(* Logix 5000 Rung export; software revision 33.00 *)

TYPE Banner_IOL_Device :
STRUCT
   Initial_Global_Read : BOOL;
   Command : SINT;
   Data : Banner_IOL_Device_Index;
   Reset : BOOL;
END_STRUCT
END_TYPE

TYPE Banner_IOL_Device_Index :
STRUCT
   Index : Banner_IOL_Device_SubIndex[39];
END_STRUCT
END_TYPE

TYPE Banner_IOL_Device_SubIndex :
STRUCT
   Sub : DINT[34];
END_STRUCT
END_TYPE

TYPE Banner_IOL_Rules :
STRUCT
   Byte_Pos : SINT;   // Byte Position to read from or write data to.
   Multi : SINT;   // Determines if a multiple byte length index is being accessed. Use 2 for 2 bytes length, 3 for 3 byte length, etc..
   BitControl : BOOL;   // 0=Standard byte contorl, 1=Bitwise packaging
   BitPos : SINT;   // Bit start position for operation
   BitValue : SINT;
   Sub_Index : SINT;
   Signed : SINT;   // 0=Unsigned, 1=Signed
END_STRUCT
END_TYPE

TYPE Banner_IOL_Rules_Array :
STRUCT
   Length : DINT;
   Settings : Banner_IOL_Rules_SettingsArray[39];
END_STRUCT
END_TYPE

TYPE Banner_IOL_Rules_SettingsArray :
STRUCT
   Index : DINT;
   Sub_Index : DINT;
   Num_Op : INT;   // Number of Operations to read/write Index.
   Total_Bytes : INT;
   RW : SINT;   // 0 = Read Only, 1 = Write Only, 2 = Read or Write
   Rules : Banner_IOL_Rules[34];   // Sub Index Position in IODD.
END_STRUCT
END_TYPE

VAR_GLOBAL   (* controller tags *)
   S4B_IOLM1_01 : Banner_IOL_Device;
        .DATA.INDEX[2]   // Direct Parameters 1 (ro)
        .DATA.INDEX[2].SUB[1]   // Reserved
        .DATA.INDEX[2].SUB[2]   // Master Cycle Time
        .DATA.INDEX[2].SUB[3]   // Min Cycle Time
        .DATA.INDEX[2].SUB[4]   // M Sequence Capability
        .DATA.INDEX[2].SUB[5]   // IO-Link Version ID
        .DATA.INDEX[2].SUB[6]   // Process Data Input Length
        .DATA.INDEX[2].SUB[7]   // Process Data Output Length
        .DATA.INDEX[2].SUB[8]   // Vendor ID
        .DATA.INDEX[2].SUB[9]   // Device ID
        .DATA.INDEX[3]   // Standard Command (wo)
        .DATA.INDEX[3].SUB[1]   // Standard Command: 126=Locator Start, 127=Locator Stop, 129=Application Reset, 164=Reset All Metrics
        .DATA.INDEX[4]   // Serial Number (ro)
        .DATA.INDEX[4].SUB[1]   // SN1
        .DATA.INDEX[4].SUB[2]   // SN2
        .DATA.INDEX[4].SUB[3]   // SN3
        .DATA.INDEX[4].SUB[4]   // SN4
        .DATA.INDEX[4].SUB[5]   // SN5
        .DATA.INDEX[4].SUB[6]   // SN6
        .DATA.INDEX[4].SUB[7]   // SN7
        .DATA.INDEX[4].SUB[8]   // SN8
        .DATA.INDEX[4].SUB[9]   // SN9
        .DATA.INDEX[4].SUB[10]   // SN10
        .DATA.INDEX[4].SUB[11]   // SN11
        .DATA.INDEX[4].SUB[12]   // SN12
        .DATA.INDEX[4].SUB[13]   // SN13
        .DATA.INDEX[4].SUB[14]   // SN14
        .DATA.INDEX[4].SUB[15]   // SN15
        .DATA.INDEX[4].SUB[16]   // SN16
        .DATA.INDEX[5]   // Configurable IO Pin Settings
        .DATA.INDEX[5].SUB[1]   // Pin Control: 0=Weak Beam, 1=Auxiliary Output, 2=Indicatoer Override Input, 3=Unused
        .DATA.INDEX[5].SUB[2]   // Control Type: 0=PNP, 1=NPN
        .DATA.INDEX[5].SUB[3]   // Indicator Override Host: 0=Enabled, 1=Disabled
        .DATA.INDEX[5].SUB[4]   // Indicator Override Guest 1: 0=Enabled, 1=Disabled
        .DATA.INDEX[5].SUB[5]   // Indicator Override Guest 2: 0=Enabled, 1=Disabled
        .DATA.INDEX[5].SUB[6]   // Indicator Override Guest 3: 0=Enabled, 1=Disabled
        .DATA.INDEX[6]   // All Curtains Clear Settings
        .DATA.INDEX[6].SUB[1]   // Endcap Color 1: 0=Green, 1=Red, 2=Yellow, 3=White, 4=Blue, 5=Magenta, 6=Cyan
        .DATA.INDEX[6].SUB[2]   // Endcap Intensity 1: 0=High, 1=Medium, 2=Low, 3=Off
        .DATA.INDEX[6].SUB[3]   // Endcap Animation Style: 0=Steady, 1=Flash, 2=Alternate
        .DATA.INDEX[6].SUB[4]   // Endcap Color 2: 0=Green, 1=Red, 2=Yellow, 3=White, 4=Blue, 5=Magenta, 6=Cyan
        .DATA.INDEX[6].SUB[5]   // Endcap Intensity 2: 0=High, 1=Medium, 2=Low, 3=Off
        .DATA.INDEX[6].SUB[6]   // Endcap Animation Speed: 0=Fast, 1=Medium, 2=Slow
        .DATA.INDEX[7]   // Any Curtain Weak Beam Settings
        .DATA.INDEX[7].SUB[1]   // Endcap Color 1: 0=Green, 1=Red, 2=Yellow, 3=White, 4=Blue, 5=Magenta, 6=Cyan
        .DATA.INDEX[7].SUB[2]   // Endcap Intensity 1: 0=High, 1=Medium, 2=Low, 3=Off
        .DATA.INDEX[7].SUB[3]   // Endcap Animation Style: 0=Steady, 1=Flash, 2=Alternate
        .DATA.INDEX[7].SUB[4]   // Endcap Color 2: 0=Green, 1=Red, 2=Yellow, 3=White, 4=Blue, 5=Magenta, 6=Cyan
        .DATA.INDEX[7].SUB[5]   // Endcap Intensity 2: 0=High, 1=Medium, 2=Low, 3=Off
        .DATA.INDEX[7].SUB[6]   // Endcap Animation Speed: 0=Fast, 1=Medium, 2=Slow
        .DATA.INDEX[8]   // This Curtain Weak Beam Settings
        .DATA.INDEX[8].SUB[1]   // Endcap Color 1: 0=Green, 1=Red, 2=Yellow, 3=White, 4=Blue, 5=Magenta, 6=Cyan
        .DATA.INDEX[8].SUB[2]   // Endcap Intensity 1: 0=High, 1=Medium, 2=Low, 3=Off
        .DATA.INDEX[8].SUB[3]   // Endcap Animation Style: 0=Steady, 1=Flash, 2=Alternate
        .DATA.INDEX[8].SUB[4]   // Endcap Color 2: 0=Green, 1=Red, 2=Yellow, 3=White, 4=Blue, 5=Magenta, 6=Cyan
        .DATA.INDEX[8].SUB[5]   // Endcap Intensity 2: 0=High, 1=Medium, 2=Low, 3=Off
        .DATA.INDEX[8].SUB[6]   // Endcap Animation Speed: 0=Fast, 1=Medium, 2=Slow
        .DATA.INDEX[9]   // Any Curtain Blocked Settings
        .DATA.INDEX[9].SUB[1]   // Endcap Color 1: 0=Green, 1=Red, 2=Yellow, 3=White, 4=Blue, 5=Magenta, 6=Cyan
        .DATA.INDEX[9].SUB[2]   // Endcap Intensity 1: 0=High, 1=Medium, 2=Low, 3=Off
        .DATA.INDEX[9].SUB[3]   // Endcap Animation Style: 0=Steady, 1=Flash, 2=Alternate
        .DATA.INDEX[9].SUB[4]   // Endcap Color 2: 0=Green, 1=Red, 2=Yellow, 3=White, 4=Blue, 5=Magenta, 6=Cyan
        .DATA.INDEX[9].SUB[5]   // Endcap Intensity 2: 0=High, 1=Medium, 2=Low, 3=Off
        .DATA.INDEX[9].SUB[6]   // Endcap Animation Speed: 0=Fast, 1=Medium, 2=Slow
        .DATA.INDEX[10]   // This Curtain Blocked Settings
        .DATA.INDEX[10].SUB[1]   // Endcap Color 1: 0=Green, 1=Red, 2=Yellow, 3=White, 4=Blue, 5=Magenta, 6=Cyan
        .DATA.INDEX[10].SUB[2]   // Endcap Intensity 1: 0=High, 1=Medium, 2=Low, 3=Off
        .DATA.INDEX[10].SUB[3]   // Endcap Animation Style: 0=Steady, 1=Flash, 2=Alternate
        .DATA.INDEX[10].SUB[4]   // Endcap Color 2: 0=Green, 1=Red, 2=Yellow, 3=White, 4=Blue, 5=Magenta, 6=Cyan
        .DATA.INDEX[10].SUB[5]   // Endcap Intensity 2: 0=High, 1=Medium, 2=Low, 3=Off
        .DATA.INDEX[10].SUB[6]   // Endcap Animation Speed: 0=Fast, 1=Medium, 2=Slow
        .DATA.INDEX[11]   // Indicator Override Input Settings
        .DATA.INDEX[11].SUB[1]   // Endcap Color 1: 0=Green, 1=Red, 2=Yellow, 3=White, 4=Blue, 5=Magenta, 6=Cyan
        .DATA.INDEX[11].SUB[2]   // Endcap Intensity 1: 0=High, 1=Medium, 2=Low, 3=Off
        .DATA.INDEX[11].SUB[3]   // Endcap Animation Style: 0=Steady, 1=Flash, 2=Alternate
        .DATA.INDEX[11].SUB[4]   // Endcap Color 2: 0=Green, 1=Red, 2=Yellow, 3=White, 4=Blue, 5=Magenta, 6=Cyan
        .DATA.INDEX[11].SUB[5]   // Endcap Intensity 2: 0=High, 1=Medium, 2=Low, 3=Off
        .DATA.INDEX[11].SUB[6]   // Endcap Animation Speed: 0=Fast, 1=Medium, 2=Slow
        .DATA.INDEX[12]   // Indicator Override IOL 1 Settings
        .DATA.INDEX[12].SUB[1]   // Endcap Color 1: 0=Green, 1=Red, 2=Yellow, 3=White, 4=Blue, 5=Magenta, 6=Cyan
        .DATA.INDEX[12].SUB[2]   // Endcap Intensity 1: 0=High, 1=Medium, 2=Low, 3=Off
        .DATA.INDEX[12].SUB[3]   // Endcap Animation Style: 0=Steady, 1=Flash, 2=Alternate
        .DATA.INDEX[12].SUB[4]   // Endcap Color 2: 0=Green, 1=Red, 2=Yellow, 3=White, 4=Blue, 5=Magenta, 6=Cyan
        .DATA.INDEX[12].SUB[5]   // Endcap Intensity 2: 0=High, 1=Medium, 2=Low, 3=Off
        .DATA.INDEX[12].SUB[6]   // Endcap Animation Speed: 0=Fast, 1=Medium, 2=Slow
        .DATA.INDEX[13]   // Indicator Override IOL 2 Settings
        .DATA.INDEX[13].SUB[1]   // Endcap Color 1: 0=Green, 1=Red, 2=Yellow, 3=White, 4=Blue, 5=Magenta, 6=Cyan
        .DATA.INDEX[13].SUB[2]   // Endcap Intensity 1: 0=High, 1=Medium, 2=Low, 3=Off
        .DATA.INDEX[13].SUB[3]   // Endcap Animation Style: 0=Steady, 1=Flash, 2=Alternate
        .DATA.INDEX[13].SUB[4]   // Endcap Color 2: 0=Green, 1=Red, 2=Yellow, 3=White, 4=Blue, 5=Magenta, 6=Cyan
        .DATA.INDEX[13].SUB[5]   // Endcap Intensity 2: 0=High, 1=Medium, 2=Low, 3=Off
        .DATA.INDEX[13].SUB[6]   // Endcap Animation Speed: 0=Fast, 1=Medium, 2=Slow
        .DATA.INDEX[14]   // Indicator Override IOL 3 Settings
        .DATA.INDEX[14].SUB[1]   // Endcap Color 1: 0=Green, 1=Red, 2=Yellow, 3=White, 4=Blue, 5=Magenta, 6=Cyan
        .DATA.INDEX[14].SUB[2]   // Endcap Intensity 1: 0=High, 1=Medium, 2=Low, 3=Off
        .DATA.INDEX[14].SUB[3]   // Endcap Animation Style: 0=Steady, 1=Flash, 2=Alternate
        .DATA.INDEX[14].SUB[4]   // Endcap Color 2: 0=Green, 1=Red, 2=Yellow, 3=White, 4=Blue, 5=Magenta, 6=Cyan
        .DATA.INDEX[14].SUB[5]   // Endcap Intensity 2: 0=High, 1=Medium, 2=Low, 3=Off
        .DATA.INDEX[14].SUB[6]   // Endcap Animation Speed: 0=Fast, 1=Medium, 2=Slow
        .DATA.INDEX[15]   // Indicator Override IOL 4 Settings
        .DATA.INDEX[15].SUB[1]   // Endcap Color 1: 0=Green, 1=Red, 2=Yellow, 3=White, 4=Blue, 5=Magenta, 6=Cyan
        .DATA.INDEX[15].SUB[2]   // Endcap Intensity 1: 0=High, 1=Medium, 2=Low, 3=Off
        .DATA.INDEX[15].SUB[3]   // Endcap Animation Style: 0=Steady, 1=Flash, 2=Alternate
        .DATA.INDEX[15].SUB[4]   // Endcap Color 2: 0=Green, 1=Red, 2=Yellow, 3=White, 4=Blue, 5=Magenta, 6=Cyan
        .DATA.INDEX[15].SUB[5]   // Endcap Intensity 2: 0=High, 1=Medium, 2=Low, 3=Off
        .DATA.INDEX[15].SUB[6]   // Endcap Animation Speed: 0=Fast, 1=Medium, 2=Slow
        .DATA.INDEX[16]   // Indicator Override IOL 5 Settings
        .DATA.INDEX[16].SUB[1]   // Endcap Color 1: 0=Green, 1=Red, 2=Yellow, 3=White, 4=Blue, 5=Magenta, 6=Cyan
        .DATA.INDEX[16].SUB[2]   // Endcap Intensity 1: 0=High, 1=Medium, 2=Low, 3=Off
        .DATA.INDEX[16].SUB[3]   // Endcap Animation Style: 0=Steady, 1=Flash, 2=Alternate
        .DATA.INDEX[16].SUB[4]   // Endcap Color 2: 0=Green, 1=Red, 2=Yellow, 3=White, 4=Blue, 5=Magenta, 6=Cyan
        .DATA.INDEX[16].SUB[5]   // Endcap Intensity 2: 0=High, 1=Medium, 2=Low, 3=Off
        .DATA.INDEX[16].SUB[6]   // Endcap Animation Speed: 0=Fast, 1=Medium, 2=Slow
        .DATA.INDEX[17]   // Indicator Override IOL 6 Settings
        .DATA.INDEX[17].SUB[1]   // Endcap Color 1: 0=Green, 1=Red, 2=Yellow, 3=White, 4=Blue, 5=Magenta, 6=Cyan
        .DATA.INDEX[17].SUB[2]   // Endcap Intensity 1: 0=High, 1=Medium, 2=Low, 3=Off
        .DATA.INDEX[17].SUB[3]   // Endcap Animation Style: 0=Steady, 1=Flash, 2=Alternate
        .DATA.INDEX[17].SUB[4]   // Endcap Color 2: 0=Green, 1=Red, 2=Yellow, 3=White, 4=Blue, 5=Magenta, 6=Cyan
        .DATA.INDEX[17].SUB[5]   // Endcap Intensity 2: 0=High, 1=Medium, 2=Low, 3=Off
        .DATA.INDEX[17].SUB[6]   // Endcap Animation Speed: 0=Fast, 1=Medium, 2=Slow
        .DATA.INDEX[18]   // Indicator Override IOL 7 Settings
        .DATA.INDEX[18].SUB[1]   // Endcap Color 1: 0=Green, 1=Red, 2=Yellow, 3=White, 4=Blue, 5=Magenta, 6=Cyan
        .DATA.INDEX[18].SUB[2]   // Endcap Intensity 1: 0=High, 1=Medium, 2=Low, 3=Off
        .DATA.INDEX[18].SUB[3]   // Endcap Animation Style: 0=Steady, 1=Flash, 2=Alternate
        .DATA.INDEX[18].SUB[4]   // Endcap Color 2: 0=Green, 1=Red, 2=Yellow, 3=White, 4=Blue, 5=Magenta, 6=Cyan
        .DATA.INDEX[18].SUB[5]   // Endcap Intensity 2: 0=High, 1=Medium, 2=Low, 3=Off
        .DATA.INDEX[18].SUB[6]   // Endcap Animation Speed: 0=Fast, 1=Medium, 2=Slow
        .DATA.INDEX[19]   // Indicator Override IOL 8 Settings
        .DATA.INDEX[19].SUB[1]   // Endcap Color 1: 0=Green, 1=Red, 2=Yellow, 3=White, 4=Blue, 5=Magenta, 6=Cyan
        .DATA.INDEX[19].SUB[2]   // Endcap Intensity 1: 0=High, 1=Medium, 2=Low, 3=Off
        .DATA.INDEX[19].SUB[3]   // Endcap Animation Style: 0=Steady, 1=Flash, 2=Alternate
        .DATA.INDEX[19].SUB[4]   // Endcap Color 2: 0=Green, 1=Red, 2=Yellow, 3=White, 4=Blue, 5=Magenta, 6=Cyan
        .DATA.INDEX[19].SUB[5]   // Endcap Intensity 2: 0=High, 1=Medium, 2=Low, 3=Off
        .DATA.INDEX[19].SUB[6]   // Endcap Animation Speed: 0=Fast, 1=Medium, 2=Slow
        .DATA.INDEX[20]   // Indicator Override IOL 9 Settings
        .DATA.INDEX[20].SUB[1]   // Endcap Color 1: 0=Green, 1=Red, 2=Yellow, 3=White, 4=Blue, 5=Magenta, 6=Cyan
        .DATA.INDEX[20].SUB[2]   // Endcap Intensity 1: 0=High, 1=Medium, 2=Low, 3=Off
        .DATA.INDEX[20].SUB[3]   // Endcap Animation Style: 0=Steady, 1=Flash, 2=Alternate
        .DATA.INDEX[20].SUB[4]   // Endcap Color 2: 0=Green, 1=Red, 2=Yellow, 3=White, 4=Blue, 5=Magenta, 6=Cyan
        .DATA.INDEX[20].SUB[5]   // Endcap Intensity 2: 0=High, 1=Medium, 2=Low, 3=Off
        .DATA.INDEX[20].SUB[6]   // Endcap Animation Speed: 0=Fast, 1=Medium, 2=Slow
        .DATA.INDEX[21]   // Fault Lockout Settings
        .DATA.INDEX[21].SUB[1]   // Endcap Color 1: 0=Green, 1=Red, 2=Yellow, 3=White, 4=Blue, 5=Magenta, 6=Cyan
        .DATA.INDEX[21].SUB[2]   // Endcap Intensity 1: 0=High, 1=Medium, 2=Low, 3=Off
        .DATA.INDEX[21].SUB[3]   // Endcap Animation Style: 0=Steady, 1=Flash, 2=Alternate
        .DATA.INDEX[21].SUB[4]   // Endcap Color 2: 0=Green, 1=Red, 2=Yellow, 3=White, 4=Blue, 5=Magenta, 6=Cyan
        .DATA.INDEX[21].SUB[5]   // Endcap Intensity 2: 0=High, 1=Medium, 2=Low, 3=Off
        .DATA.INDEX[21].SUB[6]   // Endcap Animation Speed: 0=Fast, 1=Medium, 2=Slow
        .DATA.INDEX[22]   // Lockout 1 (ro)
        .DATA.INDEX[22].SUB[1]   // Lockout Condition: 0 to 65535
        .DATA.INDEX[22].SUB[2]   // Sub Code: 0 to 65535
        .DATA.INDEX[22].SUB[3]   // Instance: 0 to 65535
        .DATA.INDEX[22].SUB[4]   // Source Module: 0=Host, 1=Guest 1, 2=Guest 2, 3=Guest 3
        .DATA.INDEX[22].SUB[5]   // Source Micro: 0=Micro A, 1=Micro B
        .DATA.INDEX[23]   // Lockout 2 (ro)
        .DATA.INDEX[23].SUB[1]   // Lockout Condition: 0 to 65535
        .DATA.INDEX[23].SUB[2]   // Sub Code: 0 to 65535
        .DATA.INDEX[23].SUB[3]   // Instance: 0 to 65535
        .DATA.INDEX[23].SUB[4]   // Source Module: 0=Host, 1=Guest 1, 2=Guest 2, 3=Guest 3
        .DATA.INDEX[23].SUB[5]   // Source Micro: 0=Micro A, 1=Micro B
        .DATA.INDEX[24]   // Lockout 3 (ro)
        .DATA.INDEX[24].SUB[1]   // Lockout Condition: 0 to 65535
        .DATA.INDEX[24].SUB[2]   // Sub Code: 0 to 65535
        .DATA.INDEX[24].SUB[3]   // Instance: 0 to 65535
        .DATA.INDEX[24].SUB[4]   // Source Module: 0=Host, 1=Guest 1, 2=Guest 2, 3=Guest 3
        .DATA.INDEX[24].SUB[5]   // Source Micro: 0=Micro A, 1=Micro B
        .DATA.INDEX[25]   // Lockout 4 (ro)
        .DATA.INDEX[25].SUB[1]   // Lockout Condition: 0 to 65535
        .DATA.INDEX[25].SUB[2]   // Sub Code: 0 to 65535
        .DATA.INDEX[25].SUB[3]   // Instance: 0 to 65535
        .DATA.INDEX[25].SUB[4]   // Source Module: 0=Host, 1=Guest 1, 2=Guest 2, 3=Guest 3
        .DATA.INDEX[25].SUB[5]   // Source Micro: 0=Micro A, 1=Micro B
        .DATA.INDEX[26]   // Lockout 5 (ro)
        .DATA.INDEX[26].SUB[1]   // Lockout Condition: 0 to 65535
        .DATA.INDEX[26].SUB[2]   // Sub Code: 0 to 65535
        .DATA.INDEX[26].SUB[3]   // Instance: 0 to 65535
        .DATA.INDEX[26].SUB[4]   // Source Module: 0=Host, 1=Guest 1, 2=Guest 2, 3=Guest 3
        .DATA.INDEX[26].SUB[5]   // Source Micro: 0=Micro A, 1=Micro B
        .DATA.INDEX[27]   // Lockout 6 (ro)
        .DATA.INDEX[27].SUB[1]   // Lockout Condition: 0 to 65535
        .DATA.INDEX[27].SUB[2]   // Sub Code: 0 to 65535
        .DATA.INDEX[27].SUB[3]   // Instance: 0 to 65535
        .DATA.INDEX[27].SUB[4]   // Source Module: 0=Host, 1=Guest 1, 2=Guest 2, 3=Guest 3
        .DATA.INDEX[27].SUB[5]   // Source Micro: 0=Micro A, 1=Micro B
        .DATA.INDEX[28]   // Lockout 7 (ro)
        .DATA.INDEX[28].SUB[1]   // Lockout Condition: 0 to 65535
        .DATA.INDEX[28].SUB[2]   // Sub Code: 0 to 65535
        .DATA.INDEX[28].SUB[3]   // Instance: 0 to 65535
        .DATA.INDEX[28].SUB[4]   // Source Module: 0=Host, 1=Guest 1, 2=Guest 2, 3=Guest 3
        .DATA.INDEX[28].SUB[5]   // Source Micro: 0=Micro A, 1=Micro B
        .DATA.INDEX[29]   // Lockout 8 (ro)
        .DATA.INDEX[29].SUB[1]   // Lockout Condition: 0 to 65535
        .DATA.INDEX[29].SUB[2]   // Sub Code: 0 to 65535
        .DATA.INDEX[29].SUB[3]   // Instance: 0 to 65535
        .DATA.INDEX[29].SUB[4]   // Source Module: 0=Host, 1=Guest 1, 2=Guest 2, 3=Guest 3
        .DATA.INDEX[29].SUB[5]   // Source Micro: 0=Micro A, 1=Micro B
        .DATA.INDEX[30]   // Lockout 9 (ro)
        .DATA.INDEX[30].SUB[1]   // Lockout Condition: 0 to 65535
        .DATA.INDEX[30].SUB[2]   // Sub Code: 0 to 65535
        .DATA.INDEX[30].SUB[3]   // Instance: 0 to 65535
        .DATA.INDEX[30].SUB[4]   // Source Module: 0=Host, 1=Guest 1, 2=Guest 2, 3=Guest 3
        .DATA.INDEX[30].SUB[5]   // Source Micro: 0=Micro A, 1=Micro B
        .DATA.INDEX[31]   // Lockout 10 (ro)
        .DATA.INDEX[31].SUB[1]   // Lockout Condition: 0 to 65535
        .DATA.INDEX[31].SUB[2]   // Sub Code: 0 to 65535
        .DATA.INDEX[31].SUB[3]   // Instance: 0 to 65535
        .DATA.INDEX[31].SUB[4]   // Source Module: 0=Host, 1=Guest 1, 2=Guest 2, 3=Guest 3
        .DATA.INDEX[31].SUB[5]   // Source Micro: 0=Micro A, 1=Micro B
        .DATA.INDEX[32]   // Host Safety Firmware Version (ro)
        .DATA.INDEX[32].SUB[1]   // Firmware 1
        .DATA.INDEX[32].SUB[2]   // Firmware 2
        .DATA.INDEX[32].SUB[3]   // Firmware 3
        .DATA.INDEX[32].SUB[4]   // Firmware 4
        .DATA.INDEX[32].SUB[5]   // Firmware 5
        .DATA.INDEX[32].SUB[6]   // Firmware 6
        .DATA.INDEX[32].SUB[7]   // Firmware 7
        .DATA.INDEX[32].SUB[8]   // Firmware 8
        .DATA.INDEX[33]   // Guest 1 Safety Firmware Version (ro)
        .DATA.INDEX[33].SUB[1]   // Firmware 1
        .DATA.INDEX[33].SUB[2]   // Firmware 2
        .DATA.INDEX[33].SUB[3]   // Firmware 3
        .DATA.INDEX[33].SUB[4]   // Firmware 4
        .DATA.INDEX[33].SUB[5]   // Firmware 5
        .DATA.INDEX[33].SUB[6]   // Firmware 6
        .DATA.INDEX[33].SUB[7]   // Firmware 7
        .DATA.INDEX[33].SUB[8]   // Firmware 8
        .DATA.INDEX[34]   // Guest 2 Safety Firmware Version (ro)
        .DATA.INDEX[34].SUB[1]   // Firmware 1
        .DATA.INDEX[34].SUB[2]   // Firmware 2
        .DATA.INDEX[34].SUB[3]   // Firmware 3
        .DATA.INDEX[34].SUB[4]   // Firmware 4
        .DATA.INDEX[34].SUB[5]   // Firmware 5
        .DATA.INDEX[34].SUB[6]   // Firmware 6
        .DATA.INDEX[34].SUB[7]   // Firmware 7
        .DATA.INDEX[34].SUB[8]   // Firmware 8
        .DATA.INDEX[35]   // Guest 3 Safety Firmware Version (ro)
        .DATA.INDEX[35].SUB[1]   // Firmware 1
        .DATA.INDEX[35].SUB[2]   // Firmware 2
        .DATA.INDEX[35].SUB[3]   // Firmware 3
        .DATA.INDEX[35].SUB[4]   // Firmware 4
        .DATA.INDEX[35].SUB[5]   // Firmware 5
        .DATA.INDEX[35].SUB[6]   // Firmware 6
        .DATA.INDEX[35].SUB[7]   // Firmware 7
        .DATA.INDEX[35].SUB[8]   // Firmware 8
        .DATA.INDEX[36]   // Number of Channels per Stick (ro)
        .DATA.INDEX[36].SUB[1]   // Number of Channels on Host
        .DATA.INDEX[36].SUB[2]   // Number of Channels on Guest 1
        .DATA.INDEX[36].SUB[3]   // Number of Channels on Guest 2
        .DATA.INDEX[36].SUB[4]   // Number of Channels on Guest 3
   S4B_Rules : Banner_IOL_Rules_Array;
        .SETTINGS[2]   // Direct Parameters 1
        .SETTINGS[2].RULES[0]   // Reserved
        .SETTINGS[2].RULES[1]   // Master Cycle Time
        .SETTINGS[2].RULES[2]   // Min Cycle Time
        .SETTINGS[2].RULES[3]   // M-Sequence Capability
        .SETTINGS[2].RULES[4]   // IO-Link ID
        .SETTINGS[2].RULES[5]   // Process Data Input Length
        .SETTINGS[2].RULES[6]   // Process Data Output Length
        .SETTINGS[2].RULES[7]   // Vendor ID
        .SETTINGS[2].RULES[8]   // Device ID
        .SETTINGS[3]   // Standard Command
        .SETTINGS[3].RULES[0]   // Standard Command
        .SETTINGS[4]   // Serial Number
        .SETTINGS[4].RULES[0]   // SN1
        .SETTINGS[4].RULES[1]   // SN2
        .SETTINGS[4].RULES[2]   // SN3
        .SETTINGS[4].RULES[3]   // SN4
        .SETTINGS[4].RULES[4]   // SN5
        .SETTINGS[4].RULES[5]   // SN6
        .SETTINGS[4].RULES[6]   // SN7
        .SETTINGS[4].RULES[7]   // SN8
        .SETTINGS[4].RULES[8]   // SN9
        .SETTINGS[4].RULES[9]   // SN10
        .SETTINGS[4].RULES[10]   // SN11
        .SETTINGS[4].RULES[11]   // SN12
        .SETTINGS[4].RULES[12]   // SN13
        .SETTINGS[4].RULES[13]   // SN14
        .SETTINGS[4].RULES[14]   // SN15
        .SETTINGS[4].RULES[15]   // SN16
        .SETTINGS[5]   // Configuration IO Pin Settings
        .SETTINGS[5].RULES[0]   // Pin Control
        .SETTINGS[5].RULES[1]   // Control Type
        .SETTINGS[5].RULES[2]   // Indicator Override Host
        .SETTINGS[5].RULES[3]   // Indicator Override Guest 1
        .SETTINGS[5].RULES[4]   // Indicator Override Guest 2
        .SETTINGS[5].RULES[5]   // Indicator Override Guest 3
        .SETTINGS[6]   // All Curtains Clear Settings
        .SETTINGS[6].RULES[0]   // Endcap Color 1
        .SETTINGS[6].RULES[1]   // Endcap Intensity 1
        .SETTINGS[6].RULES[2]   // Endcap Animation Style
        .SETTINGS[6].RULES[3]   // Endcap Color 2
        .SETTINGS[6].RULES[4]   // Endcap Intensity 2
        .SETTINGS[6].RULES[5]   // Endcap Animation Speed
        .SETTINGS[7]   // Any Curtain Weak Beam Settings
        .SETTINGS[7].RULES[0]   // Endcap Color 1
        .SETTINGS[7].RULES[1]   // Endcap Intensity 1
        .SETTINGS[7].RULES[2]   // Endcap Animation Style
        .SETTINGS[7].RULES[3]   // Endcap Color 2
        .SETTINGS[7].RULES[4]   // Endcap Intensity 2
        .SETTINGS[7].RULES[5]   // Endcap Animation Speed
        .SETTINGS[8]   // This Curtain Weak Beam Settings
        .SETTINGS[8].RULES[0]   // Endcap Color 1
        .SETTINGS[8].RULES[1]   // Endcap Intensity 1
        .SETTINGS[8].RULES[2]   // Endcap Animation Style
        .SETTINGS[8].RULES[3]   // Endcap Color 2
        .SETTINGS[8].RULES[4]   // Endcap Intensity 2
        .SETTINGS[8].RULES[5]   // Endcap Animation Speed
        .SETTINGS[9]   // Any Curtain Blocked Settings
        .SETTINGS[9].RULES[0]   // Endcap Color 1
        .SETTINGS[9].RULES[1]   // Endcap Intensity 1
        .SETTINGS[9].RULES[2]   // Endcap Animation Style
        .SETTINGS[9].RULES[3]   // Endcap Color 2
        .SETTINGS[9].RULES[4]   // Endcap Intensity 2
        .SETTINGS[9].RULES[5]   // Endcap Animation Speed
        .SETTINGS[10]   // This Curtain Blocked Settings
        .SETTINGS[10].RULES[0]   // Endcap Color 1
        .SETTINGS[10].RULES[1]   // Endcap Intensity 1
        .SETTINGS[10].RULES[2]   // Endcap Animation Style
        .SETTINGS[10].RULES[3]   // Endcap Color 2
        .SETTINGS[10].RULES[4]   // Endcap Intensity 2
        .SETTINGS[10].RULES[5]   // Endcap Animation Speed
        .SETTINGS[11]   // Indicator Override Input Settings
        .SETTINGS[11].RULES[0]   // Endcap Color 1
        .SETTINGS[11].RULES[1]   // Endcap Intensity 1
        .SETTINGS[11].RULES[2]   // Endcap Animation Style
        .SETTINGS[11].RULES[3]   // Endcap Color 2
        .SETTINGS[11].RULES[4]   // Endcap Intensity 2
        .SETTINGS[11].RULES[5]   // Endcap Animation Speed
        .SETTINGS[12]   // Indicator Override IOL 1 Settings
        .SETTINGS[12].RULES[0]   // Endcap Color 1
        .SETTINGS[12].RULES[1]   // Endcap Intensity 1
        .SETTINGS[12].RULES[2]   // Endcap Animation Style
        .SETTINGS[12].RULES[3]   // Endcap Color 2
        .SETTINGS[12].RULES[4]   // Endcap Intensity 2
        .SETTINGS[12].RULES[5]   // Endcap Animation Speed
        .SETTINGS[13]   // Indicator Override IOL 2 Settings
        .SETTINGS[13].RULES[0]   // Endcap Color 1
        .SETTINGS[13].RULES[1]   // Endcap Intensity 1
        .SETTINGS[13].RULES[2]   // Endcap Animation Style
        .SETTINGS[13].RULES[3]   // Endcap Color 2
        .SETTINGS[13].RULES[4]   // Encap Intensity 2
        .SETTINGS[13].RULES[5]   // Encap Animation Speed
        .SETTINGS[14]   // Indicator Override IOL 3 Settings
        .SETTINGS[14].RULES[0]   // Endcap Color 1
        .SETTINGS[14].RULES[1]   // Endcap Intensity 1
        .SETTINGS[14].RULES[2]   // Endcap Animation Style
        .SETTINGS[14].RULES[3]   // Endcap Color 2
        .SETTINGS[14].RULES[4]   // Endcap Intensity 2
        .SETTINGS[14].RULES[5]   // Endcap Animation Speed
        .SETTINGS[15]   // Indicator Override IOL 4 Settings
        .SETTINGS[15].RULES[0]   // Endcap Color 1
        .SETTINGS[15].RULES[1]   // Endcap Intensity 1
        .SETTINGS[15].RULES[2]   // Endcap Animation Style
        .SETTINGS[15].RULES[3]   // Endcap Color 2
        .SETTINGS[15].RULES[4]   // Endcap Intensity 2
        .SETTINGS[15].RULES[5]   // Endcap Animation Speed
        .SETTINGS[16]   // Indicator Override IOL 5 Settings
        .SETTINGS[16].RULES[0]   // Endcap Color 1
        .SETTINGS[16].RULES[1]   // Endcap Intensity 1
        .SETTINGS[16].RULES[2]   // Endcap Animation Style
        .SETTINGS[16].RULES[3]   // Endcap Color 2
        .SETTINGS[16].RULES[4]   // Endcap Intensity 2
        .SETTINGS[16].RULES[5]   // Endcap Animation Speed
        .SETTINGS[17]   // Indicator Override IOL 6 Settings
        .SETTINGS[17].RULES[0]   // Endcap Color 1
        .SETTINGS[17].RULES[1]   // Endcap Intensity 1
        .SETTINGS[17].RULES[2]   // Endcap Animation Style
        .SETTINGS[17].RULES[3]   // Endcap Color 2
        .SETTINGS[17].RULES[4]   // Endcap Intensity 2
        .SETTINGS[17].RULES[5]   // Endcap Animation Speed
        .SETTINGS[18]   // Indicator Override IOL 7 Settings
        .SETTINGS[18].RULES[0]   // Endcap Color 1
        .SETTINGS[18].RULES[1]   // Endcap Intensity 1
        .SETTINGS[18].RULES[2]   // Endcap Animation Style
        .SETTINGS[18].RULES[3]   // Endcap Color 2
        .SETTINGS[18].RULES[4]   // Endcap Intensity 2
        .SETTINGS[18].RULES[5]   // Endcap Animation Speed
        .SETTINGS[19]   // Indicator Override IOL 8 Settings
        .SETTINGS[19].RULES[0]   // Endcap Color 1
        .SETTINGS[19].RULES[1]   // Endcap Intensity 1
        .SETTINGS[19].RULES[2]   // Endcap Animation Style
        .SETTINGS[19].RULES[3]   // Endcap Color 2
        .SETTINGS[19].RULES[4]   // Endcap Intensity 2
        .SETTINGS[19].RULES[5]   // Endcap Animation Speed
        .SETTINGS[20]   // Indicator Override IOL 9 Settings
        .SETTINGS[20].RULES[0]   // Endcap Color 1
        .SETTINGS[20].RULES[1]   // Endcap Intensity 1
        .SETTINGS[20].RULES[2]   // Endcap Animation Style
        .SETTINGS[20].RULES[3]   // Endcap Color 2
        .SETTINGS[20].RULES[4]   // Endcap Intensity 2
        .SETTINGS[20].RULES[5]   // Endcap Animation Speed
        .SETTINGS[21]   // Fault Lockout Settings
        .SETTINGS[21].RULES[0]   // Endcap Color 1
        .SETTINGS[21].RULES[1]   // Endcap Intensity 1
        .SETTINGS[21].RULES[2]   // Endcap Animation Style
        .SETTINGS[21].RULES[3]   // Endcap Color 2
        .SETTINGS[21].RULES[4]   // Endcap Intensity 2
        .SETTINGS[21].RULES[5]   // Endcap Animation Speed
        .SETTINGS[22]   // Lockout 1
        .SETTINGS[22].RULES[0]   // Lockout Condition
        .SETTINGS[22].RULES[1]   // Sub Code
        .SETTINGS[22].RULES[2]   // Instance
        .SETTINGS[22].RULES[3]   // Source Module
        .SETTINGS[22].RULES[4]   // Source Micro
        .SETTINGS[23]   // Lockout 2
        .SETTINGS[23].RULES[0]   // Lockout Condition
        .SETTINGS[23].RULES[1]   // Sub Code
        .SETTINGS[23].RULES[2]   // Instance
        .SETTINGS[23].RULES[3]   // Source Module
        .SETTINGS[23].RULES[4]   // Source Micro
        .SETTINGS[24]   // Lockout 3
        .SETTINGS[24].RULES[0]   // Lockout Condition
        .SETTINGS[24].RULES[1]   // Sub Code
        .SETTINGS[24].RULES[2]   // Instance
        .SETTINGS[24].RULES[3]   // Source Module
        .SETTINGS[24].RULES[4]   // Source Micro
        .SETTINGS[25]   // Lockout 4
        .SETTINGS[25].RULES[0]   // Lockout Condition
        .SETTINGS[25].RULES[1]   // Sub Code
        .SETTINGS[25].RULES[2]   // Instance
        .SETTINGS[25].RULES[3]   // Source Module
        .SETTINGS[25].RULES[4]   // Source Micro
        .SETTINGS[26]   // Lockout 5
        .SETTINGS[26].RULES[0]   // Lockout Condition
        .SETTINGS[26].RULES[1]   // Sub Code
        .SETTINGS[26].RULES[2]   // Instance
        .SETTINGS[26].RULES[3]   // Source Module
        .SETTINGS[26].RULES[4]   // Source Micro
        .SETTINGS[27]   // Lockout 6
        .SETTINGS[27].RULES[0]   // Lockout Condition
        .SETTINGS[27].RULES[1]   // Sub Code
        .SETTINGS[27].RULES[2]   // Instance
        .SETTINGS[27].RULES[3]   // Source Module
        .SETTINGS[27].RULES[4]   // Source Micro
        .SETTINGS[28]   // Lockout 7
        .SETTINGS[28].RULES[0]   // Lockout Condition
        .SETTINGS[28].RULES[1]   // Sub Code
        .SETTINGS[28].RULES[2]   // Instance
        .SETTINGS[28].RULES[3]   // Source Module
        .SETTINGS[28].RULES[4]   // Source Micro
        .SETTINGS[29]   // Lockout 8
        .SETTINGS[29].RULES[0]   // Lockout Condition
        .SETTINGS[29].RULES[1]   // Sub Code
        .SETTINGS[29].RULES[2]   // Instance
        .SETTINGS[29].RULES[3]   // Source Module
        .SETTINGS[29].RULES[4]   // Source Micro
        .SETTINGS[30]   // Lockout 9
        .SETTINGS[30].RULES[0]   // Lockout Condition
        .SETTINGS[30].RULES[1]   // Sub Code
        .SETTINGS[30].RULES[2]   // Instance
        .SETTINGS[30].RULES[3]   // Source Module
        .SETTINGS[30].RULES[4]   // Source Micro
        .SETTINGS[31]   // Lockout 10
        .SETTINGS[31].RULES[0]   // Lockout Condition
        .SETTINGS[31].RULES[1]   // Sub Code
        .SETTINGS[31].RULES[2]   // Instance
        .SETTINGS[31].RULES[3]   // Source Module
        .SETTINGS[31].RULES[4]   // Source Micro
        .SETTINGS[32]   // Host Safety Firmware Version
        .SETTINGS[32].RULES[0]   // Firmware 1
        .SETTINGS[32].RULES[1]   // Firmware 2
        .SETTINGS[32].RULES[2]   // Firmware 3
        .SETTINGS[32].RULES[3]   // Firmware 4
        .SETTINGS[32].RULES[4]   // Firmware 5
        .SETTINGS[32].RULES[5]   // Firmware 6
        .SETTINGS[32].RULES[6]   // Firmware 7
        .SETTINGS[32].RULES[7]   // Firmware 8
        .SETTINGS[33]   // Guest 1 Safety Firmware Version
        .SETTINGS[33].RULES[0]   // Firmware 1
        .SETTINGS[33].RULES[1]   // Firmware 2
        .SETTINGS[33].RULES[2]   // Firmware 3
        .SETTINGS[33].RULES[3]   // Firmware 4
        .SETTINGS[33].RULES[4]   // Firmware 5
        .SETTINGS[33].RULES[5]   // Firmware 6
        .SETTINGS[33].RULES[6]   // Firmware 7
        .SETTINGS[33].RULES[7]   // Firmware 8
        .SETTINGS[34]   // Guest 2 Safety Firmware Version
        .SETTINGS[34].RULES[0]   // Firmware 1
        .SETTINGS[34].RULES[1]   // Firmware 2
        .SETTINGS[34].RULES[2]   // Firmware 3
        .SETTINGS[34].RULES[3]   // Firmware 4
        .SETTINGS[34].RULES[4]   // Firmware 5
        .SETTINGS[34].RULES[5]   // Firmware 6
        .SETTINGS[34].RULES[6]   // Firmware 7
        .SETTINGS[34].RULES[7]   // Firmware 8
        .SETTINGS[35]   // Guest 3 Safety Firmware Version
        .SETTINGS[35].RULES[0]   // Firmware 1
        .SETTINGS[35].RULES[1]   // Firmware 2
        .SETTINGS[35].RULES[2]   // Firmware 3
        .SETTINGS[35].RULES[3]   // Firmware 4
        .SETTINGS[35].RULES[4]   // Firmware 5
        .SETTINGS[35].RULES[5]   // Firmware 6
        .SETTINGS[35].RULES[6]   // Firmware 7
        .SETTINGS[35].RULES[7]   // Firmware 8
        .SETTINGS[36]   // Number of Channels per Stick
        .SETTINGS[36].RULES[0]   // Number of Channels on Host
        .SETTINGS[36].RULES[1]   // Number of Channels on Guest 1
        .SETTINGS[36].RULES[2]   // Number of Channels on Guest 2
        .SETTINGS[36].RULES[3]   // Number of Channels on Guest 3
END_VAR

PROGRAM MainProgram

ROUTINE MainRoutine   (* ladder *)
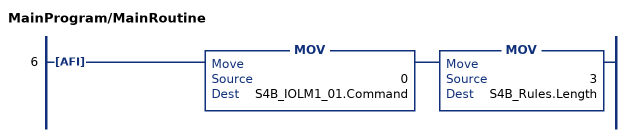
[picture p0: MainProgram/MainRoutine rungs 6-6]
   6: AFI()MOV(0,S4B_IOLM1_01.Command)MOV(3,S4B_Rules.Length);
END_ROUTINE
END_PROGRAM
